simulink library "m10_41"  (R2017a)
settings: Solver=VariableStepAuto  StartTime=0.0  StopTime=10.0  RelTol=1e-3
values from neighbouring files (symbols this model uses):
  beta = 5    [ini_mst.m]    (also in vdpini.m = sqrt(3))
  omega = 4    [ini_mst.m]    (also in vdpini.m = 1)
  x01 = 50    [ini_mst.m]
  x02 = 0    [ini_mst.m]

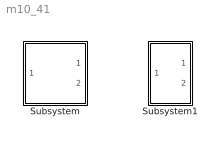
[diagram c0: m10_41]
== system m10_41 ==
  Subsystem : Subsystem
  Subsystem1 : Subsystem

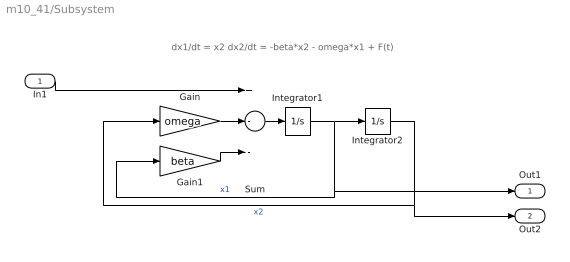
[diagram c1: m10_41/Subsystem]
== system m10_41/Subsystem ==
  note: dx1/dt = x2 dx2/dt = -beta*x2 - omega*x1 + F(t)
  In1 : Inport
  Gain : Gain  Gain=omega
  Gain1 : Gain  Gain=beta
  Integrator1 : Integrator  InitialCondition=x01
  Integrator2 : Integrator  InitialCondition=x02
  Sum : Sum  Inputs=+--
  Out1 : Outport
  Out2 : Outport  Port=2
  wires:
  In1/1 -> Sum/1
  Integrator1/1 -> Integrator2/1, Gain1/1, Out1/1  "x1"
  Gain1/1 -> Sum/3
  Sum/1 -> Integrator1/1
  Integrator2/1 -> Gain/1, Out2/1  "x2"
  Gain/1 -> Sum/2

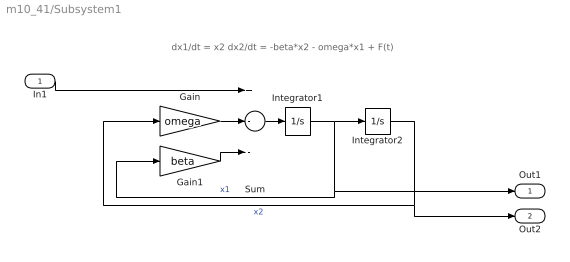
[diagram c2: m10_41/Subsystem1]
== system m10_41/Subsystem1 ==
  note: dx1/dt = x2 dx2/dt = -beta*x2 - omega*x1 + F(t)
  In1 : Inport
  Gain : Gain  Gain=omega
  Gain1 : Gain  Gain=beta
  Integrator1 : Integrator  InitialCondition=x01
  Integrator2 : Integrator  InitialCondition=x02
  Sum : Sum  Inputs=+--
  Out1 : Outport
  Out2 : Outport  Port=2
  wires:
  In1/1 -> Sum/1
  Integrator1/1 -> Integrator2/1, Gain1/1, Out1/1  "x1"
  Gain1/1 -> Sum/3
  Sum/1 -> Integrator1/1
  Integrator2/1 -> Gain/1, Out2/1  "x2"
  Gain/1 -> Sum/2
